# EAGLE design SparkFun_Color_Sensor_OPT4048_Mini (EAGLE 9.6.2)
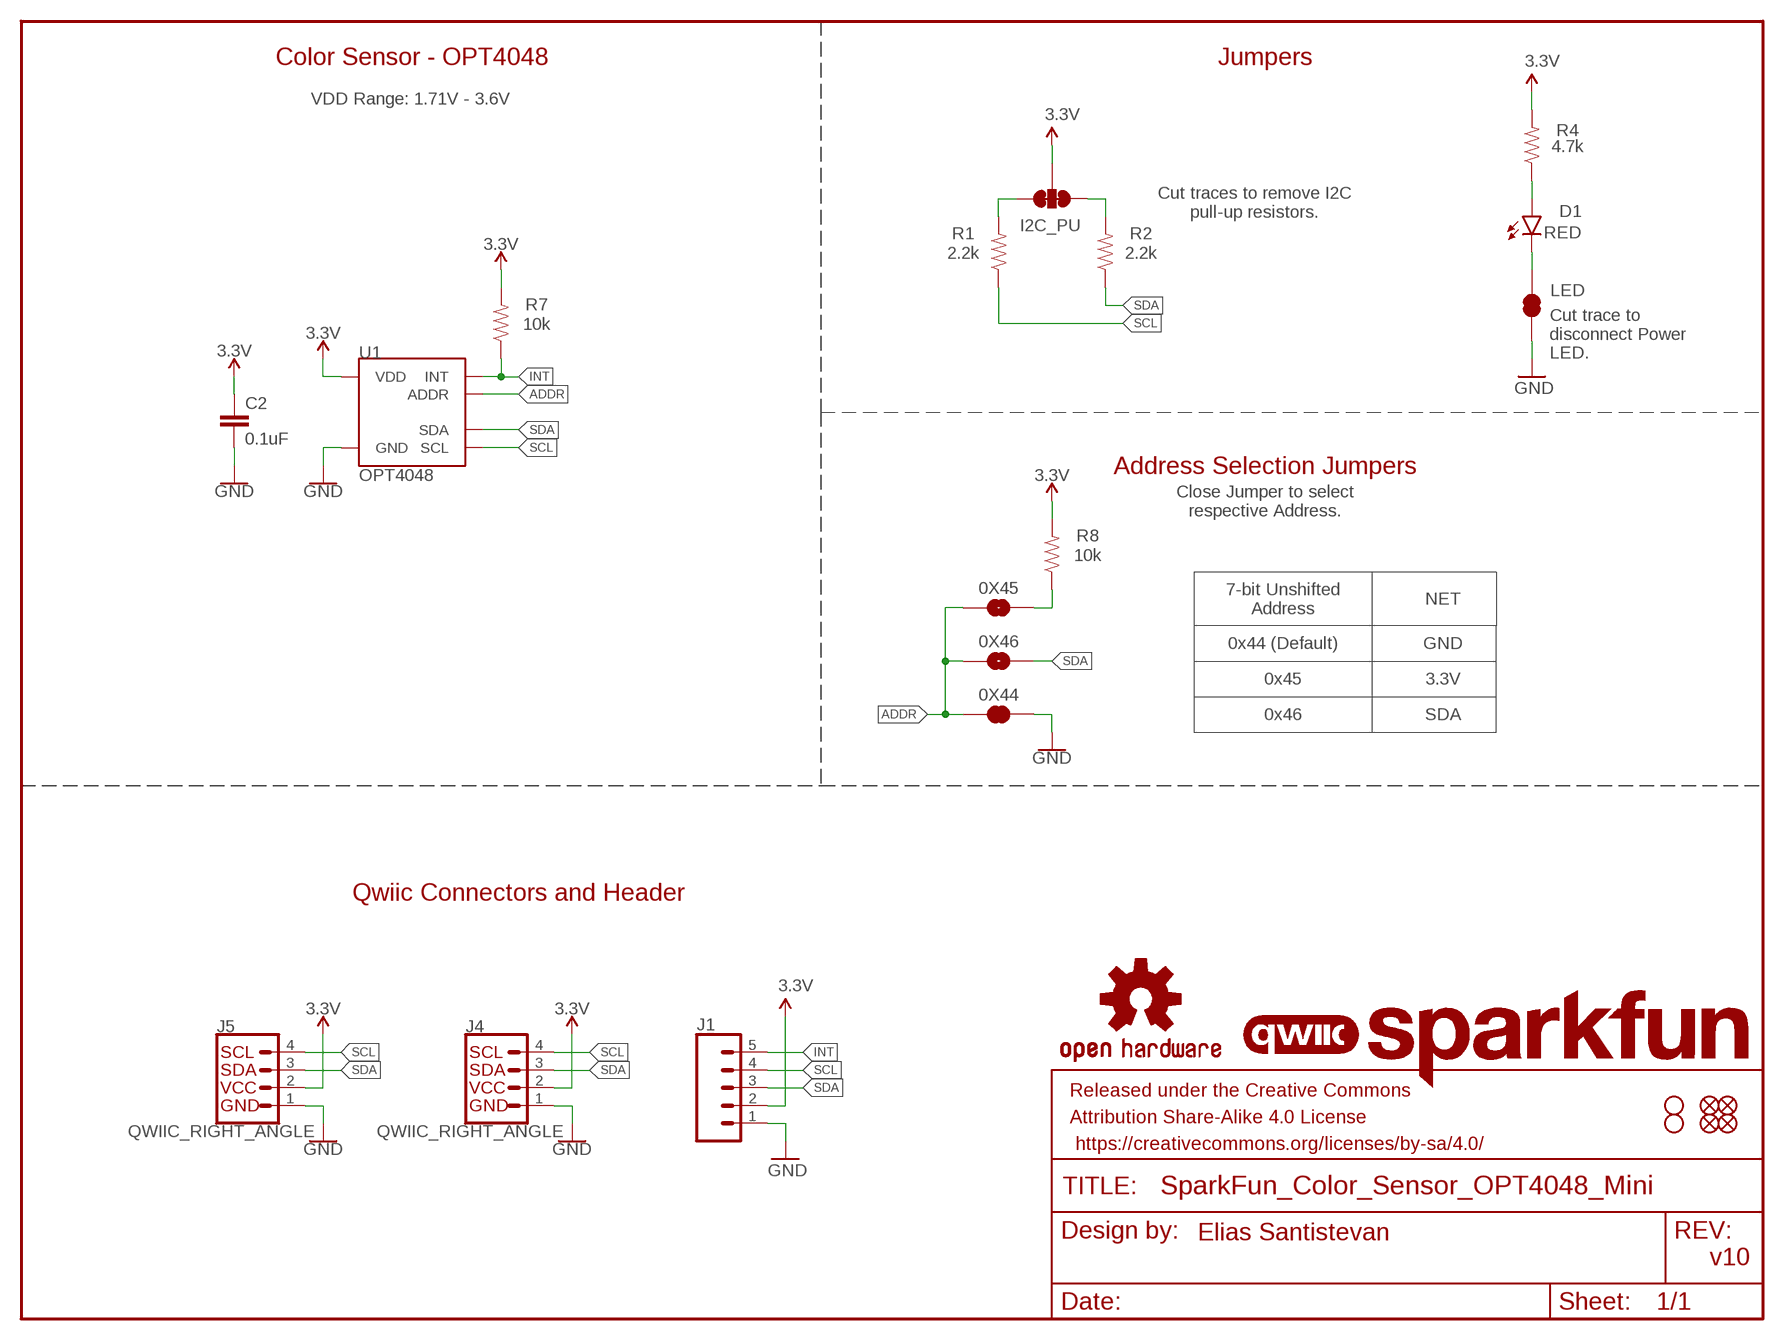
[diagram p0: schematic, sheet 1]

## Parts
0X44  JUMPER-SMT_2_NC_TRACE_SILK  [SMT-JUMPER_2_NC_TRACE_SILK]
0X45  JUMPER-SMT_2_NO_SILK  [SMT-JUMPER_2_NO_SILK]
0X46  JUMPER-SMT_2_NO_SILK  [SMT-JUMPER_2_NO_SILK]
C2  0.1uF  0.1UF-0402T-16V-10%  [0402-TIGHT]
D1  RED  LED-RED_0603-KB  [LED-0603]
FD5  FIDUCIALUFIDUCIAL  [FIDUCIAL-MICRO]
FD6  FIDUCIALUFIDUCIAL  [FIDUCIAL-MICRO]
FD7  FIDUCIALUFIDUCIAL  [FIDUCIAL-MICRO]
FD8  FIDUCIALUFIDUCIAL  [FIDUCIAL-MICRO]
FRAME2  FRAME-LETTER  [CREATIVE_COMMONS]
H7  STAND-OFFTIGHT  [STAND-OFF-TIGHT]
H8  STAND-OFFTIGHT  [STAND-OFF-TIGHT]
I2C_PU  S_MODE  JUMPER-SMT_3_2-NC_TRACE_SILK  [SMT-JUMPER_3_2-NC_TRACE_SILK]
J1  CONN_05NO_SILK  [1X05_NO_SILK]
J4  QWIIC_RIGHT_ANGLE  QWIIC_CONNECTORJS-1MM  [JST04_1MM_RA]
J5  QWIIC_RIGHT_ANGLE  QWIIC_CONNECTORJS-1MM  [JST04_1MM_RA]
LED  JUMPER-SMT_2_NC_TRACE_SILK  [SMT-JUMPER_2_NC_TRACE_SILK]
LOGO1  SFE_LOGO_NAMEBLANK  [BLANK]
LOGO2  QWIIC_LOGO_3MM  [QWIIC_3MM]
LOGO3  OSHW-LOGONO_SILK  [DUMMY]
R1  2.2k  2.2KOHM-0603-1/10W-1%  [0603]
R2  2.2k  2.2KOHM-0603-1/10W-1%  [0603]
R4  4.7k  4.7KOHM-0603-1/10W-1%  [0603]
R7  10k  10KOHM-0603-1/10W-1%  [0603]
R8  10k  10KOHM-0603-1/10W-1%  [0603]
U1  OPT4048  [FCSOT]

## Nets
3.3V: C2.1 I2C_PU.2 J1.2 J4.2 J5.2 R4.2 R7.2 R8.2 U1.P1(VDD)
ADDR: 0X44.1 0X45.1 0X46.1 U1.P2(ADDR)
GND: 0X44.2 C2.2 J1.1 J4.1 J5.1 LED.1 U1.P4(GND)
INT: J1.5 R7.1 U1.P7(INT)
N$1: I2C_PU.1 R1.2
N$2: I2C_PU.3 R2.2
N$3: D1.A R4.1
N$4: D1.C LED.2
N$9: 0X45.2 R8.1
SCL: J1.4 J4.4 J5.4 R1.1 U1.P5(SCL)
SDA: 0X46.2 J1.3 J4.3 J5.3 R2.1 U1.P8(SDA)

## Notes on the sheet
- Color Sensor - OPT4048 | Jumpers
- VDD Range: 1.71V - 3.6V
- Cut traces to remove I2C
  pull-up resistors.
- Cut trace to
  disconnect Power
  LED.
- Address Selection Jumpers
- Close Jumper to select
  respective Address.
- 7-bit Unshifted
  Address
- NET
- 0x44 (Default) | GND
- 0x45 | 3.3V
- 0x46 | SDA
- Qwiic Connectors and Header
- Elias Santistevan
- v10

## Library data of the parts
0X44 LED = SparkFun-Jumpers:JUMPER-SMT_2_NC_TRACE: Normally closed trace jumper
0X45 0X46 = SparkFun-Jumpers:JUMPER-SMT_2_NO: Normally open jumper
C2 = SparkFun-Capacitors:0.1UF: 0.1µF ceramic capacitors; PROD_ID: CAP-12416
D1 = SparkFun-LED:LED-RED: Red SMD LED; PROD_ID: DIO-17976
FD5-FD8 = SparkFun-Aesthetics:FIDUCIAL: Fiducial Alignment Points
FRAME2 = SparkFun-Aesthetics:FRAME-LETTER: Schematic Frame - Letter
H7 H8 = SparkFun-Hardware:STAND-OFF: Stand Off
I2C_PU = SparkFun-Jumpers:JUMPER-SMT_3_2-NC_TRACE: Normally closed trace jumper (2 of 2 connections) This jumper has a trace between all three pads so they are normally closed (NC). Use a razor knife to open the connection(s). For best results follow the IPC guidelines for cutting traces: Cutout at least 0.063 mm (0.005 in). Remove all loose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
J1 = SparkFun-Connectors:CONN_05: Multi connection point. Often used as Generic Header-pin footprint for 0.1 inch spaced/style header connections On any of the 0.1 inch spaced packages, you can populate with these: Break Away Headers - Straight (PRT-00116) Break Away Male Headers - Right Angle (PRT-00553) Female Headers (PRT-00115)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
J4 J5 = SparkFun-Connectors:QWIIC_CONNECTOR: SparkFun I2C Standard Qwiic Connector An SMD 1mm pitch JST connector makes it easy and quick (get it? Qwiic?) to connect I2C devices to each other. The Qwiic system enables fast and solderless connection between popular platforms and various sensors and actuators. We carry 200mm, 100mm, 50mm, and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; PROD_ID: CONN-13694
LOGO1 = SparkFun-Aesthetics:SFE_LOGO_NAME: SparkFun Font Logo
LOGO2 = SparkFun-Aesthetics:QWIIC_LOGO: Qwiic Logos for placement on schematic and PCB. The 5.5mm silk logo is best for placing next to Qwiic connector.
LOGO3 = SparkFun-Aesthetics:OSHW-LOGO: Open-Source Hardware (OSHW) Logo
R1 R2 = SparkFun-Resistors:2.2KOHM: 2.2kΩ resistor; PROD_ID: RES-08272
R4 = SparkFun-Resistors:4.7KOHM: 4.7kΩ resistor; PROD_ID: RES-07857
R7 R8 = SparkFun-Resistors:10KOHM: 10kΩ resistor; PROD_ID: RES-00824
U1 = Color_Sensor:OPT4048: Texas Instruments - OPT4048 Tristiumulus XYZ Color Sensor The OPT4048 is a single-chip high resolution color sensor, capable of measuring four channels each with specific engineered spectral responses. Three of the four channels closely match the CIE tristimulus spectra with the fourth channel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; PROD_ID: IC-18868

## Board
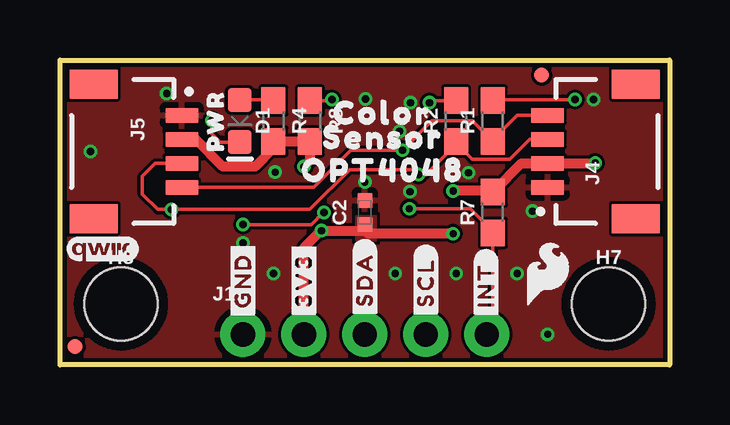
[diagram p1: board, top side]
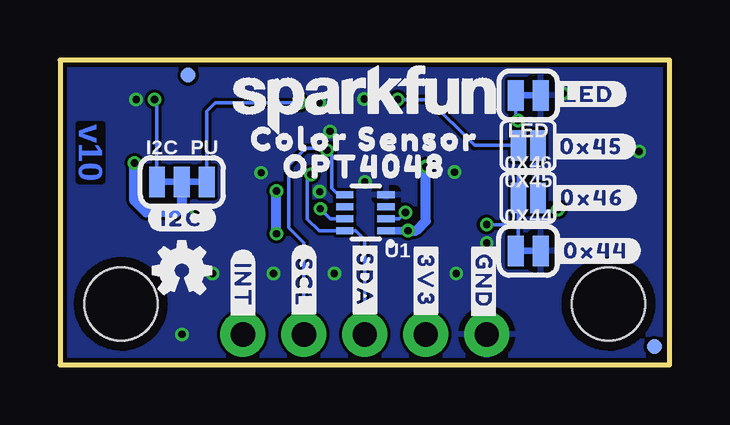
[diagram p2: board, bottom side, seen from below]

Size 25.4 x 12.7 mm. Coordinates in mm from the lower left corner, seen from the top.
Outline: 0,0 0,12.7 25.4,12.7 25.4,0 0,0
Copper layers (1*16): Top 0.035mm / dielectric 1.5mm / Bottom 0.035mm
Design rules "SparkFun-2-Layer-Minimum-JLCPCB": minimum track width 5mil, minimum drill 0.3mm, track to track 5mil, track to pad 5mil, pad to pad 5mil, via to via 5mil, smd to smd 5mil, copper to edge 7mil, drill to drill 7mil, minimum pad ring 5mil, minimum via ring 5mil, stop-mask expansion 2.5mil, vias tented up to drill 25mil, thermal gap 10mil

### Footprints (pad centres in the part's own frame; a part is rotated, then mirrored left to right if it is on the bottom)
SMT-JUMPER_2_NC_TRACE_SILK = smd 0.66 x 1.27: 1 -0.521,0; 2 0.521,0
SMT-JUMPER_2_NO_SILK = smd 0.635 x 1.27: 1 -0.406,0; 2 0.406,0
0402-TIGHT = smd 0.6 x 0.6: 1 -0.5,0; 2 0.5,0
LED-0603 = smd 1 x 1: A -0.877,0; C 0.877,0
FIDUCIAL-MICRO = smd 0.635 x 0.635: 1 0,0
STAND-OFF-TIGHT = hole 3.048: 0,0
SMT-JUMPER_3_2-NC_TRACE_SILK = smd 0.66 x 1.27: 1 -1.041,0; 2 0,0; 3 1.041,0
1X05_NO_SILK = drill 1.016 pad 1.88: 1 0,0; 2 2.54,0; 3 5.08,0; 4 7.62,0; 5 10.16,0
JST04_1MM_RA = smd 0.6 x 1.35: 1 -1.5,0; 2 -0.5,0; 3 0.5,0; 4 1.5,0 | smd 1.2 x 2: NC1 2.8,-3.675; NC2 -2.8,-3.675
0603 = smd 1.1 x 1: 1 -0.85,0; 2 0.85,0
FCSOT = smd 0.72 x 0.3: P1 -0.889,0.762; P2 -0.889,0.262; P3 -0.889,-0.238; P4 -0.889,-0.738; P5 0.831,-0.738; P6 0.831,-0.238; P7 0.831,0.262; P8 0.831,0.762

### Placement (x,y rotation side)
0X44  5.89,4.75 0 bottom
0X45  5.89,9.14 180 bottom
0X46  5.89,6.96 0 bottom
C2  12.7,6.35 90 top
D1  7.49,10.16 270 top
FD5  20.07,12.06 0 bottom
FD6  0.64,0.76 0 bottom
FD7  0.64,0.76 0 top
FD8  20.07,12.06 0 top
FRAME2  not placed on the board
H7  22.86,2.54 0 top
H8  2.54,2.54 0 top
I2C_PU  20.32,7.62 0 bottom
J1  7.62,1.27 0 top
J4  20.32,8.89 90 top
J5  5.08,8.89 270 top
LED  5.89,11.23 180 bottom
LOGO1  not placed on the board
LOGO2  1.78,4.83 0 top
LOGO3  not placed on the board
LOGO4  SPECIAL_INSTRUCTIONS-ORDERING  [ORDERING_INSTRUCTIONS]  not placed on the board
R1  18.03,10.16 90 top
R2  16.51,10.16 90 top
R4  8.89,10.16 270 top
R7  18.03,6.35 90 top
R8  10.41,10.16 270 top
U1  12.7,6.35 180 bottom
U$1  [#INT#9]  17.75,3.33 90 top
U$2  [COLOR_SENSOR227]  12.7,9.4 0 bottom
U$3  [OPT4048229]  12.7,8.26 0 bottom
U$4  [#0X44#11]  3.07,4.75 0 bottom
U$5  [#0X46#11]  3.23,6.96 0 bottom
U$6  [#0X45#11]  3.25,9.09 0 bottom
U$7  [#INT#3]  17.78,3.3 270 bottom
U$8  [SFE_LOGO_NAME_.1]  12.7,11.05 0 bottom
U$9  [COLOR14]  13.44,10.49 0 top
U$10  [#3V3#0]  10.16,3.51 270 bottom
U$11  [SENSOR15]  13.46,9.47 0 top
U$12  [OPT4048229]  13.46,8.1 0 top
U$13  [#SDA#1]  12.7,3.53 270 bottom
U$14  [#LED#11]  3.38,11.28 0 bottom
U$15  [OSHW-LOGO-MINI]  20.32,3.94 0 bottom
U$16  [#GND#4]  7.75,3.48 270 bottom
U$19  [#SCL#5]  15.24,3.43 270 bottom
U$20  [#I2C#11]  20.32,6.1 0 bottom
U$35  [SFE_LOGO_FLAME_.1]  20.32,3.81 0 top
U$37  [#3V3#0]  10.16,3.51 90 top
U$38  [#GND#4]  7.62,3.51 90 top
U$39  [#SCL#5]  15.24,3.43 90 top
U$40  [#SDA#6]  12.7,3.56 90 top
U$43  [PWR8821882023]  6.48,10.16 90 top

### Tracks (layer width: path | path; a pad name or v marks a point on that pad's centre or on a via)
3.3V  (via drill 0.3)
  Top 0.406: J1.2 10.16,4.88 10.87,5.59 v10.9,5.59 12.84,5.59 12.84,5.46 v16.38,5.46 | R7.2 18.12,7.28 | 18.12,7.28 19.22,8.39 J4.2 22.28,8.39 v22.3,8.41 | v16.38,7.24 16.43,7.28 18.12,7.28 | v10.16,8.26 10.41,8.51 R8.2 R4.2 8.89,9.02 8.13,8.26 6.78,8.26 5.65,9.39 J5.2
  Bottom 0.305: U1.P1 v10.9,5.59
  Bottom 0.406: v16.38,5.46 v16.38,7.24 | I2C_PU.2 20.32,6.58 20.55,6.35 21.82,6.35 22.3,6.83 v22.3,8.41 | v10.9,5.59 10.57,5.59 10.16,5.99 v10.16,8.26
  pour Top (no thermals): 12.34,6.1 12.34,5.21 13.16,5.21 13.16,6.17 12.34,6.17 12.34,6.12
ADDR  (via drill 0.3)
  Top 0.152: v11,6.35 10.97,6.35 10.46,5.84 v7.62,5.84
  Bottom 0.152: U1.P2 11.26,6.09 v11,6.35 | 0X44.1 6.3,4.86 6.3,5.82 | 6.3,5.82 0X46.1 6.3,7.87 6.12,8.05 5.9,8.05 5.49,8.46 0X45.1 | v7.62,5.84 6.33,5.84 6.3,5.82
GND  (via drill 0.3)
  other vias: 13.97,3.81 8.89,3.81 7.62,5.08 14.61,10.92 22.23,11.05 17.02,8 14.58,7.21 14.15,9.73 1.27,8.89 20.32,1.27 12.73,11.07 16.51,3.81 19.05,3.81 12.7,7.62 4.45,11.3 19.68,6.4 8.97,8.03
  pour Top (rank 4): 0,12.7 25.4,12.7 25.4,0 0,0
  pour Bottom (rank 4): 0,12.7 25.4,12.7 25.4,0 0,0
INT  (via drill 0.3)
  Top 0.152: v14.55,6.5 17.09,6.5 18.03,5.56 R7.1 18.03,1.52 J1.5
  Bottom 0.152: U1.P7 14.14,6.09 v14.55,6.5
N$1  (via drill 0.3)
  Top 0.152: v21.46,11.05 18.07,11.05 R1.2
  Bottom 0.152: I2C_PU.1 21.36,10.95 v21.46,11.05
N$2  (via drill 0.3)
  Top 0.152: v15.39,10.92 15.48,11.01 R2.2
  Bottom 0.152: I2C_PU.3 19.28,10.57 18.92,10.92 v15.39,10.92
N$3
  Top 0.152: D1.A 8.89,11.04
  Top 0.406: 8.89,11.04 R4.1
N$4  (via drill 0.3)
  Top 0.152: v6.33,10.19 6.33,9.63 6.67,9.28 D1.C
  Bottom 0.152: LED.2 6.41,10.27 v6.33,10.19
N$9  (via drill 0.3)
  Top 0.152: v11.33,11.05 11.29,11.01 R8.1
  Bottom 0.152: v11.33,11.05 10.03,11.05 8.13,9.14 0X45.2
SCL  (via drill 0.3)
  Top 0.152: J4.4 19.05,10.39 18.82,10.16 18.03,9.37 R1.1 17.2,10.15 17.2,10.16 15.49,10.16 v14.28,8.94 12.12,8.94 10.56,7.39 J5.4
  Bottom 0.152: U1.P5 13.55,7.11 13.82,7.11 14.07,7.37 14.07,8.74 v14.28,8.94 14.35,9.02 15.16,9.02 15.88,8.31 15.88,5.71 15.24,5.08 J1.4
SDA  (via drill 0.3)
  Top 0.152: J4.3 19.58,9.39 18.75,8.56 17.17,8.56 16.51,9.22 R2.1 16.51,9.19 15.24,7.92 v14.94,7.92 14.73,8.13 12.06,8.13 10.41,6.48 v4.65,6.48 4.06,6.48 3.43,7.11 3.43,7.85 3.97,8.39 J5.3
  Bottom 0.152: v14.94,7.92 15.09,7.77 15.09,6.07 14.61,5.59 U1.P8 13.08,5.59 12.7,5.21 J1.3 | 0X46.2 5.49,6.55 5.33,6.4 4.72,6.4 v4.65,6.48

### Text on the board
Bottom: v10
Measures: Units in Inches
tDocu: 1.6mm Thickness / 1 oz. Copper / Lead-Free HASL finish / Material: TG135-140 / Red Soldermask / White Silkscreen | Elias Santistevan

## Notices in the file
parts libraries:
SparkFun-Aesthetics: Licensing: Creative Commons ShareAlike 4.0 International - https://creativecommons.org/licenses/by-sa/4.0
SparkFun-Aesthetics: Released under the Creative Commons Attribution Share-Alike 4.0 License
SparkFun-Aesthetics: https://creativecommons.org/licenses/by-sa/4.0
